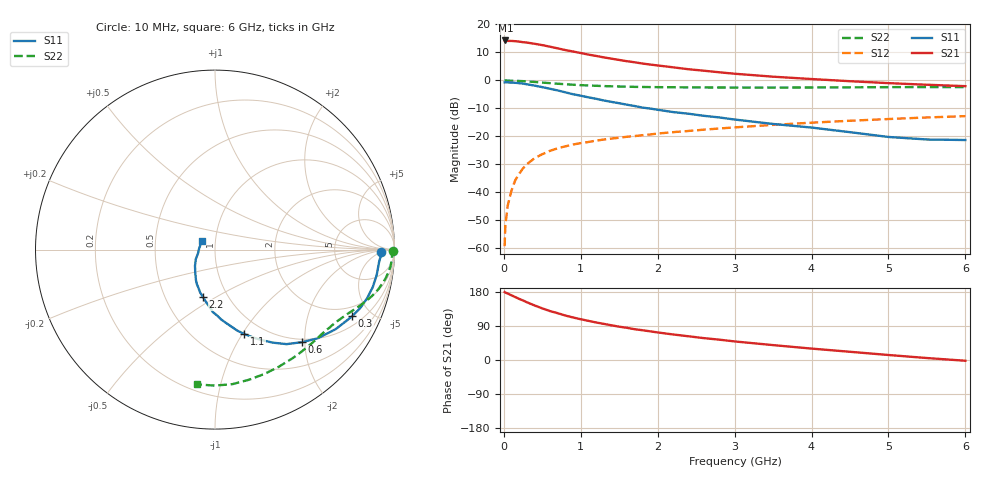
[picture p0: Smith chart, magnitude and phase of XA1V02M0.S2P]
! SIEMENS Discrete & RF Semiconductors
! BFY180
! Si NPN RF Bipolar Junction Transistor in MICRO-X
! VCE = 1 V  IC = 2 mA
! Common Emitter S-Parameters:  May  1997
# GHz  S  MA  R  50
!  f  S11  S21  S12  S22
! GHz  MAG  ANG  MAG  ANG  MAG  ANG  MAG  ANG
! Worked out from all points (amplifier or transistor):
!   36 points, 10 MHz to 6 GHz, reference 50 ohm
!   highest |S21| = 14.2 dB at 20 MHz (marker M1)
!   |S21| within 3 dB of that: start of sweep to 730 MHz
!   unconditionally stable (mu >= 1): 1.613 GHz to end of sweep
!   at 250 MHz: K = 0.20, MSG = 22.5 dB, |S12| = -31.4 dB
!   at 1.4 GHz: K = 0.93, MSG = 14.3 dB, |S12| = -20.8 dB
!   at 6 GHz: K = 1.21, MAG = 2.6 dB, |S12| = -12.8 dB
!   S11 on the Smith chart (normalised r, x): 10 MHz: 24, -4; 300 MHz: 1.43, -3.84; 600 MHz: 0.94, -1.94; 1.1 GHz: 0.82, -1.02; 2.2 GHz: 0.77, -0.44; 6 GHz: 0.86, +0.08
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0.01  0.9222 -0.7  5.039 179.3  0.0011 83.0  0.989 -0.4
0.02  0.9257 -1.8  5.144 178.0  0.0026 89.4  0.9999 -0.8
0.05  0.9167 -4.4  5.049 175.4  0.0058 86.9  0.9875 -1.9
0.1  0.912 -8.9  5.04 170.7  0.0109 85.4  0.9854 -3.8
0.15  0.9035 -13.4  4.991 165.9  0.0167 81.2  0.9821 -5.6
0.2  0.8899 -17.7  4.906 161.2  0.0215 79.2  0.9737 -7.4
0.3  0.8503 -25.9  4.716 152.3  0.0319 74.0  0.9558 -10.8
0.4  0.8048 -33.5  4.486 143.9  0.0409 69.4  0.9353 -13.8
0.5  0.7554 -40.9  4.247 136.2  0.0481 65.1  0.9117 -16.5
0.6  0.7076 -46.8  3.98 129.1  0.0552 62.0  0.8902 -18.7
0.8  0.6107 -58.1  3.465 117.3  0.0664 56.5  0.8515 -22.6
1  0.5314 -66.8  3.066 107.5  0.0758 52.7  0.8204 -25.9
1.1  0.4966 -71.0  2.877 103.3  0.0794 51.1  0.8092 -27.4
1.3  0.4369 -78.2  2.565 95.3  0.0878 49.1  0.7896 -30.3
1.5  0.3903 -85.0  2.311 87.9  0.0947 47.4  0.7754 -33.2
1.7  0.3483 -92.0  2.1 81.3  0.1012 45.9  0.7641 -36.0
2.2  0.2716 -104.3  1.707 67.4  0.119 42.4  0.7518 -43.1
3  0.1999 -122.1  1.311 49.0  0.1447 37.1  0.7438 -54.2
3.5  0.1666 -131.4  1.161 39.3  0.1604 33.7  0.7432 -61.2
4.5  0.1188 -153.9  0.964 21.7  0.1901 25.9  0.7494 -75.2
5.5  0.088 173.4  0.834 5.2  0.2176 17.5  0.7577 -90.1
6  0.0861 147.6  0.787 -2.0  0.2297 13.1  0.7577 -97.6
